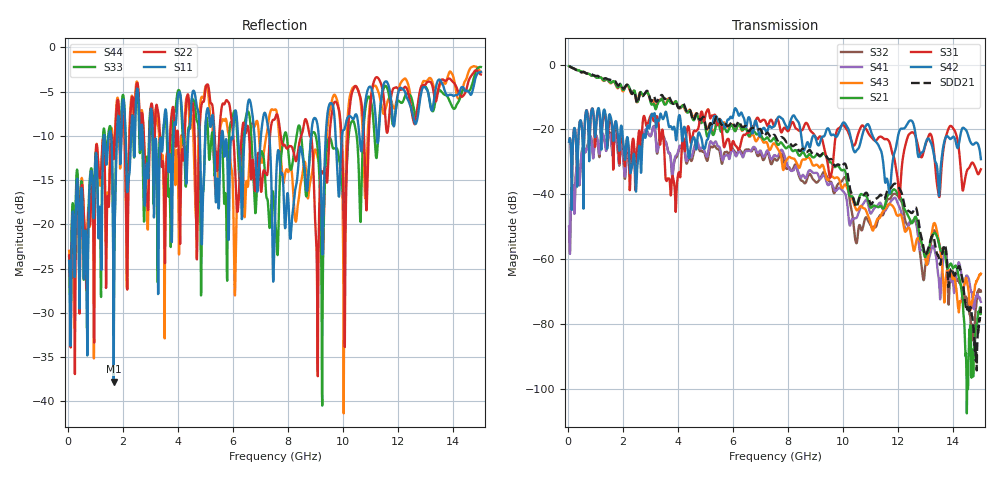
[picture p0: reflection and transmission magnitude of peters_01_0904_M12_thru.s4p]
# MHZ S RI R 50.00
! FREQ  S11  S12  S13  S14
!  S21  S22  S23  S24
!  S31  S32  S33  S34
!  S41  S42  S43  S44
!  REAL  IMAG  REAL  IMAG  REAL  IMAG  REAL  IMAG
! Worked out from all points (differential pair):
!   1496 points, 50 MHz to 15 GHz, reference 50 ohm
!   strongest paths, dB at 50 MHz, 3.79 GHz, 7.53 GHz, 11.27 GHz, 15 GHz:
!     S42: -23.8, -19.9, -18.6, -24.7, -29.2
!     S31: -23.8, -34.6, -18.2, -22.6, -32.3
!     S21: -0.5, -11.9, -23.1, -44.0, -75.7
!     S43: -0.5, -11.8, -24.6, -47.4, -64.4
!     S41: -49.9, -34.4, -28.0, -43.1, -73.1
!     S32: -50.2, -34.2, -29.1, -47.7, -69.9
!   taken as a pair (ports 1,3 in; 2,4 out), SDD21 dB: -0.5, -11.8, -22.0, -40.9, -74.6
!   lowest |S11| = -37.8 dB at 1.67 GHz (marker M1), VSWR 1.03, Z = 50.2 - j1.28 ohm
!   |S11| at or under -10 dB: start of sweep to 1.309 GHz; 3.088 GHz to 3.466 GHz (377.7 MHz wide, 11.5 % of centre); 7.318 GHz to 8.837 GHz (1.518 GHz wide, 18.8 % of centre)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
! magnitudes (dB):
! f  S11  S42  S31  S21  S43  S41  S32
! 50 MHz  -24.1  -23.8  -23.8  -0.5  -0.5  -49.9  -50.2
! 1.67 GHz  -37.8  -23.0  -27.2  -5.1  -5.2  -24.9  -25.1
! 3.91 GHz  -8.8  -21.8  -43.6  -11.3  -11.4  -28.2  -28.9
! 5.07 GHz  -6.9  -23.2  -14.0  -22.2  -20.0  -28.3  -29.7
! 9.05 GHz  -8.5  -24.2  -23.0  -27.7  -30.9  -33.4  -36.4
! 11.88 GHz  -8.1  -26.7  -29.9  -38.6  -45.0  -41.0  -39.8
! 15 GHz  -2.8  -29.2  -32.3  -75.7  -64.4  -73.1  -69.9
